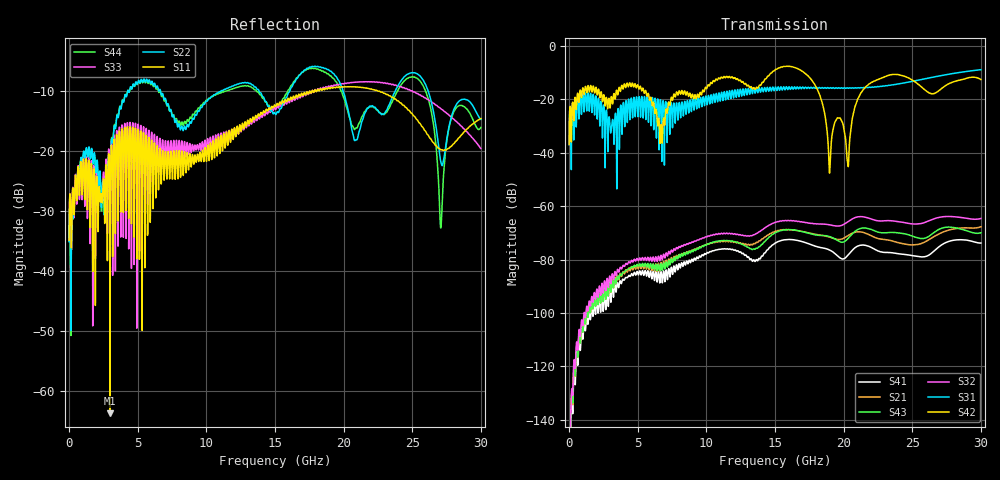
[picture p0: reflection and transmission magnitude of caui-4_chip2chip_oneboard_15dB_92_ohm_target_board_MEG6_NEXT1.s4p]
! Touchstone file from project caui-4_chip2chip_oneboard
! Exported from Circuit Design 8.0.0
! Variables:
!  $ModelNames_Index = 0
!  $ModelNames_Index1 = 0
!  $ModelNames_Index2 = 0
!  $ModelNames_Index3 = 0
!  $ModelNames_Index4 = 0
!  $ModelNames_Index5 = 0
!  Lbo = 0.5in
!  Lmain = 16in
!  lcap = 0.25in
# GHZ S MA R 50.000000
! Modal data exported
! Port[1] = Port1
! Port[2] = Port2
! Port[3] = Port3
! Port[4] = Port4
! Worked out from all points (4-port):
!   3000 points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, 10 MHz to 30 GHz, reference 50 ohm
!   strongest paths, dB at 10 MHz, 7.51 GHz, 15.01 GHz, 22.51 GHz, 30 GHz:
!     S42: -36.9, -20.0, -9.0, -12.6, -12.6
!     S31: -36.9, -26.7, -15.7, -15.2, -8.9
!     S32: -165.6, -76.9, -66.1, -65.5, -64.7
!     S43: -173.6, -80.8, -70.0, -69.7, -70.0
!     S21: -174.2, -80.1, -69.4, -72.2, -67.7
!     S41: -185.9, -84.5, -73.9, -76.8, -73.8
!   lowest |S11| = -63.7 dB at 2.99 GHz (marker M1), VSWR 1.00, Z = 50 + j0.0563 ohm
!   |S11| at or under -10 dB: start of sweep to 17.7 GHz; 17.77 GHz to 17.88 GHz (110.5 MHz wide, 0.62 % of centre); 22.48 GHz to end of sweep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
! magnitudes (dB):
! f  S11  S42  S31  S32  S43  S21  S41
! 10 MHz  -34.9  -36.9  -36.9  -165.6  -173.6  -174.2  -185.9
! 2.99 GHz  -63.7  -23.3  -30.1  -86.5  -89.4  -88.6  -91.7
! 16.31 GHz  -11.0  -7.9  -16.2  -65.5  -68.9  -69.0  -72.6
! 20.3 GHz  -9.3  -43.9  -15.8  -65.9  -72.3  -71.2  -78.6
! 22.09 GHz  -9.7  -13.6  -15.4  -65.0  -68.9  -71.3  -75.7
! 27.08 GHz  -19.8  -16.2  -11.1  -64.1  -68.4  -70.1  -74.7
! 30 GHz  -14.6  -12.6  -8.9  -64.7  -70.0  -67.7  -73.8
